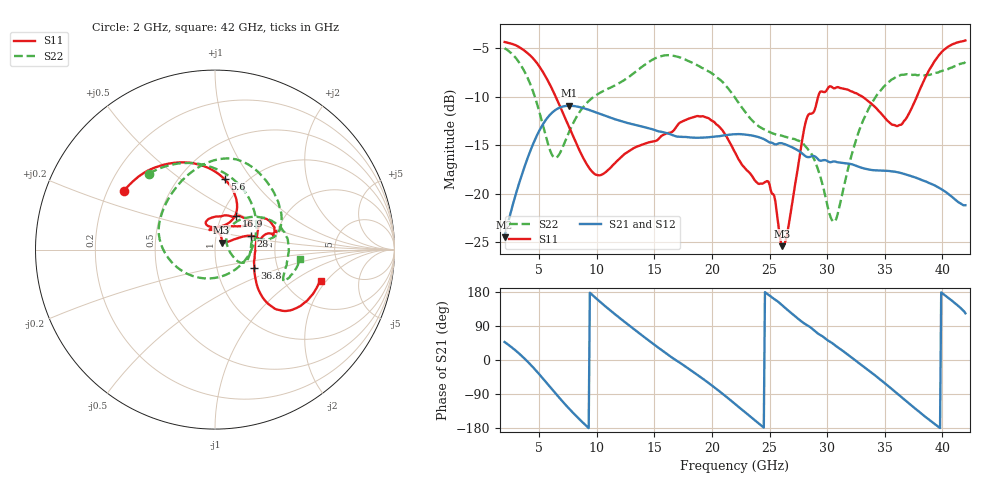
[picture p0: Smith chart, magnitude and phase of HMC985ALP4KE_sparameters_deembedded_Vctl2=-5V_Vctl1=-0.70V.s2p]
!s2p File: Measurements: S11, S21, S12, S22
# GHz S dB R 50.0
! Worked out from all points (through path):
!   401 points, 2 GHz to 42 GHz, reference 50 ohm
!   highest |S21| = -10.94 dB at 7.6 GHz (marker M1); lowest = -24.5 dB at 2 GHz (marker M2)
!   lowest |S11| = -25.4 dB at 26.1 GHz (marker M3), VSWR 1.11, Z = 53.6 + j4.23 ohm
!   |S11| at or under -10 dB: 6.429 GHz to 29.22 GHz (22.79 GHz wide, 128 % of centre); 33.05 GHz to 37.79 GHz (4.743 GHz wide, 13.4 % of centre)
!   |S22| runs from -22.9 to -5.0 dB; largest |S21 - S12| = 0.00029
!   S11 on the Smith chart (normalised r, x): 2 GHz: 0.27, +0.27; 5.6 GHz: 0.80, +0.75; 16.9 GHz: 1.17, +0.46; 28 GHz: 1.48, +0.24; 36.8 GHz: 1.52, -0.33; 42 GHz: 3.10, -1.76
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2  -4.39 147.4  -24.47 47.5  -24.47 47.5  -5.02 131.0
3.6  -5.17 120.8  -17.67 7.5  -17.68 7.5  -7.15 85.9
4.7  -6.39 99.9  -14.27 -27.0  -14.27 -27.0  -10.30 44.2
5.6  -8.03 82.3  -12.36 -58.6  -12.37 -58.6  -14.18 -5.3
6.5  -10.18 67.8  -11.31 -91.0  -11.32 -90.9  -16.27 -75.7
7.6  -13.15 59.3  -10.94 -128.5  -10.95 -128.5  -13.63 -140.9
8.7  -16.03 64.7  -11.14 -162.5  -11.14 -162.5  -11.26 -173.6
11.9  -16.47 109.4  -12.45 113.0  -12.46 113.0  -8.65 139.8
15.4  -14.32 77.7  -13.59 31.4  -13.59 31.4  -5.91 86.4
16.9  -13.13 58.1  -14.10 -1.1  -14.10 -1.0  -5.86 68.6
19.6  -12.17 35.2  -14.20 -58.2  -14.20 -58.2  -7.34 32.3
22  -15.73 52.7  -13.87 -115.9  -13.88 -115.8  -10.10 11.1
24.9  -18.74 99.8  -14.66 172.0  -14.66 172.1  -13.60 12.2
26.1  -25.39 47.0  -14.81 144.2  -14.82 144.2  -14.04 -1.0
28  -13.33 21.0  -16.03 96.6  -16.03 96.7  -14.96 -23.6
28.7  -11.73 11.2  -16.12 82.7  -16.13 82.7  -16.02 -27.0
30.7  -9.13 19.0  -16.68 38.4  -16.69 38.5  -22.81 24.8
32.9  -9.91 32.5  -17.29 -11.5  -17.30 -11.5  -13.11 49.6
35.4  -12.65 10.2  -17.66 -71.2  -17.66 -71.1  -8.46 20.9
36.8  -12.35 -24.9  -18.00 -106.8  -18.01 -106.7  -7.71 3.7
39.6  -5.92 -42.4  -19.31 -175.0  -19.31 -175.0  -7.53 -24.3
42  -4.23 -16.7  -21.18 123.3  -21.19 123.3  -6.44 -6.2
